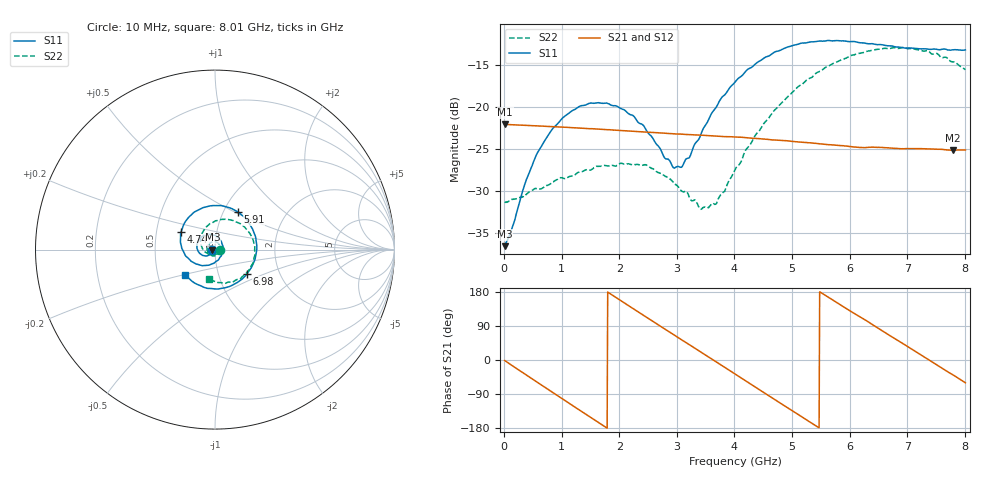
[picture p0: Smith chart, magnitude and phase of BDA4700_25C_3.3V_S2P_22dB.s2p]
!Agilent Technologies,E5071B,MY42404982,A.09.10
!Date: Mon Oct 20 18:12:18 2025
!Data & Calibration Information:
!Freq	S11:SOLT2(ON)	S21:SOLT2(ON)	S12:SOLT2(ON)	S22:SOLT2(ON)
# Hz S RI R 50
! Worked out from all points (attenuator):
!   801 points, 10 MHz to 8.01 GHz, reference 50 ohm
!   highest |S21| = -22.07 dB at 20 MHz (marker M1); lowest = -25.2 dB at 7.79 GHz (marker M2)
!   lowest |S11| = -36.6 dB at 10 MHz (marker M3), VSWR 1.03, Z = 48.5 - j0.12 ohm
!   |S11| at or under -10 dB: start of sweep to end of sweep
!   |S22| runs from -32.2 to -13.0 dB; largest |S21 - S12| = 0.0009
!   S11 on the Smith chart (normalised r, x): 10 MHz: 0.97, -0.00; 4.74 GHz: 0.67, +0.14; 5.91 GHz: 1.16, +0.52; 6.98 GHz: 1.37, -0.39; 8.01 GHz: 0.69, -0.21
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1e7  -0.0148 -0.00124  0.0788 -0.0017  0.0788 -0.00175  0.0271 -0.0008
2e7  -0.0152 -0.00196  0.0787 -0.00297  0.0787 -0.00325  0.027 -0.00111
5.9e8  -0.0414 -0.0348  0.0384 -0.0667  0.0384 -0.0667  0.0137 -0.0295
1e9  -0.0809 -0.0245  -0.0146 -0.0743  -0.0146 -0.0743  -0.015 -0.0348
1.35e9  -0.1011 0.0105  -0.0538 -0.0517  -0.0538 -0.0518  -0.037 -0.0179
2.07e9  -0.0468 0.0843  -0.064 0.0333  -0.064 0.0333  -0.0303 0.0344
2.68e9  0.0339 0.0475  -0.00321 0.07  -0.00333 0.0699  0.0143 0.0381
2.94e9  0.0431 0.00588  0.0266 0.0637  0.0266 0.0636  0.0265 0.0237
3.08e9  0.0397 -0.0183  0.0409 0.0552  0.0403 0.0555  0.0291 0.0124
3.41e9  0.00395 -0.0672  0.0631 0.0251  0.0631 0.0251  0.0212 -0.0126
3.54e9  -0.0182 -0.0803  0.0666 0.0105  0.0667 0.0104  0.0137 -0.0211
3.69e9  -0.0492 -0.0871  0.0666 -0.00653  0.0666 -0.00673  0.000789 -0.0267
4.01e9  -0.1201 -0.072  0.0529 -0.0397  0.053 -0.0396  -0.0325 -0.0269
4.74e9  -0.189 0.0991  -0.0199 -0.0602  -0.0195 -0.0603  -0.0804 0.057
5.35e9  -0.0609 0.2352  -0.0594 -0.0132  -0.0593 -0.0135  -0.0157 0.1489
5.91e9  0.1265 0.2111  -0.044 0.0386  -0.0441 0.0383  0.1115 0.1569
6.35e9  0.2201 0.0863  -0.00801 0.057  -0.00793 0.0566  0.1978 0.0841
6.68e9  0.227 -0.0355  0.023 0.0521  0.0231 0.0521  0.2213 -0.00248
6.98e9  0.1773 -0.1355  0.0444 0.0349  0.0444 0.0346  0.2061 -0.083
7.41e9  0.0385 -0.2159  0.0561 -0.00289  0.0561 -0.00296  0.1243 -0.1665
7.79e9  -0.1018 -0.1924  0.0429 -0.0347  0.0428 -0.0348  0.0189 -0.1839
8.01e9  -0.1647 -0.1422  0.0276 -0.048  0.0277 -0.048  -0.0339 -0.1622
